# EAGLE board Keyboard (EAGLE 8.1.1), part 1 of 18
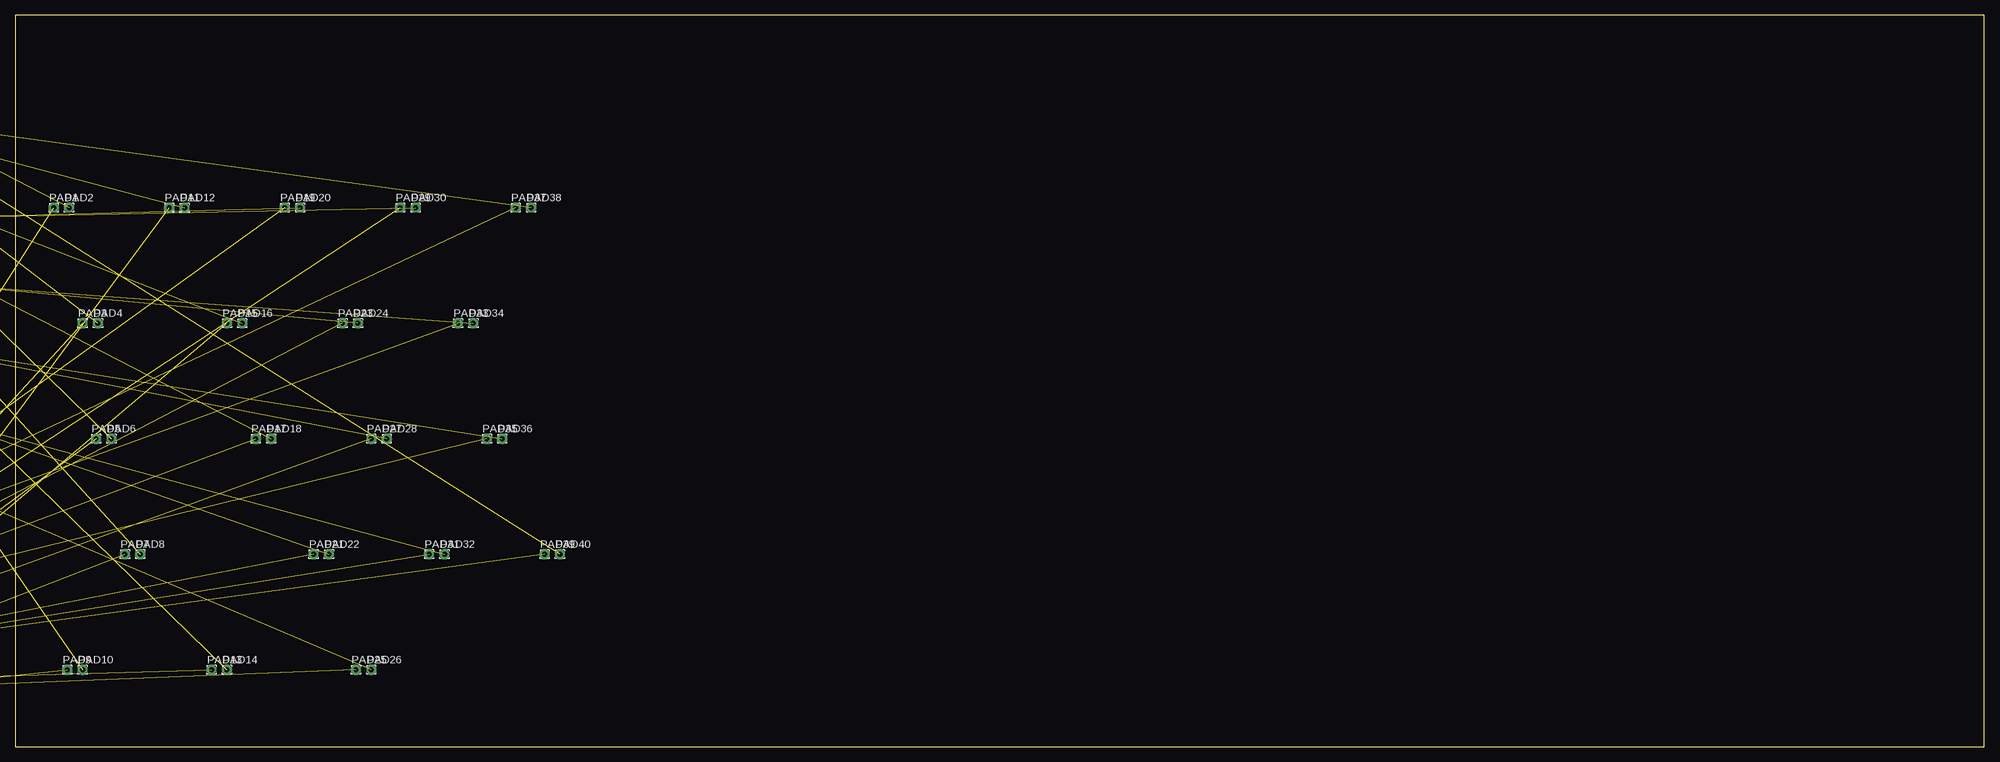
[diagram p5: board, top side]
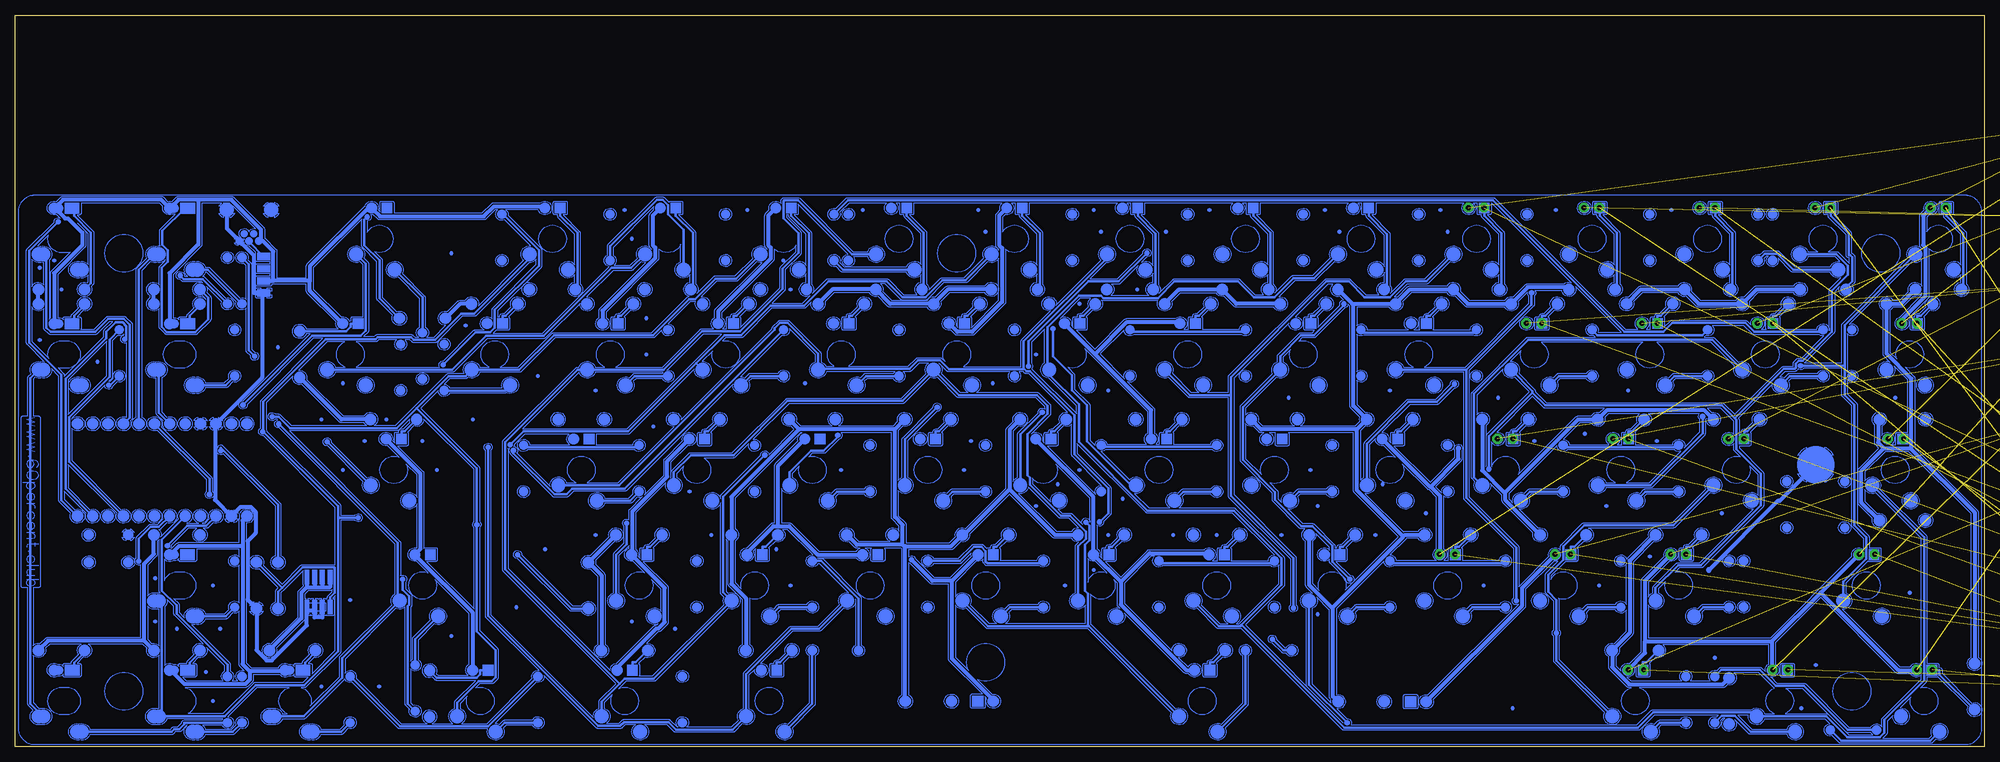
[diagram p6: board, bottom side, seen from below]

Size 324.79 x 120.64 mm. Coordinates in mm from the lower left corner, seen from the top.
Outline: 0,0 324.79,0 324.79,120.64 0,120.64 0,0
Copper layers (1*16): Top 0.035mm / dielectric 1.5mm / Bottom 0.035mm
Design rules "default": minimum track width 10mil, minimum drill 24mil, track to track 8mil, track to pad 8mil, pad to pad 8mil, via to via 8mil, smd to smd 8mil, copper to edge 40mil, drill to drill 8mil, minimum pad ring 10mil, minimum via ring 8mil, stop-mask expansion 4mil, vias tented up to drill 0mil, thermal gap 10mil

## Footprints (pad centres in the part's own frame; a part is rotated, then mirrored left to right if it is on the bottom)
2X5-SHROUDED = drill 1.016 pad 1.88: 1 -1.27,5.08; 2 1.27,5.08; 3 -1.27,2.54; 4 1.27,2.54; 5 -1.27,0; 6 1.27,0; 7 -1.27,-2.54; 8 1.27,-2.54; 9 -1.27,-5.08; 10 1.27,-5.08
1,6/0,8 = drill 0.813 pad 1.6 octagon: 1 0,0
R0805 = smd 1.3 x 1.5: 1 -0.95,0; 2 0.95,0
SOIC127P1030X265-20N = smd 1.981 x 0.559: 1 -4.674,5.715; 2 -4.674,4.445; 3 -4.674,3.175; 4 -4.674,1.905; 5 -4.674,0.635; 6 -4.674,-0.635; 7 -4.674,-1.905; 8 -4.674,-3.175; 9 -4.674,-4.445; 10 -4.674,-5.715; 11 4.674,-5.715; 12 4.674,-4.445; 13 4.674,-3.175; 14 4.674,-1.905; 15 4.674,-0.635; 16 4.674,0.635; 17 4.674,1.905; 18 4.674,3.175; 19 4.674,4.445; 20 4.674,5.715
SO14 = smd 0.6 x 1.2: 1 -3.81,-2.8; 2 -2.54,-2.8; 3 -1.27,-2.8; 4 0,-2.8; 5 1.27,-2.8; 6 2.54,-2.8; 7 3.81,-2.8; 8 3.81,2.8; 9 2.54,2.8; 10 1.27,2.8; 11 0,2.8; 12 -1.27,2.8; 13 -2.54,2.8; 14 -3.81,2.8
TEENSY_3.5/3.6 = drill 0.965: 0/RX -25.4,-7.62; 1/TX -22.86,-7.62; 2 -20.32,-7.62; 3/CANTX -17.78,-7.62; 3V3 7.62,-7.62; 3V3_2 17.78,-2.54; 3V3_LO -22.86,7.62; 4/CANRX -15.24,-7.62; 5 -12.7,-7.62; 6 -10.16,-7.62; 7 -7.62,-7.62; 8 -5.08,-7.62; 9/CS -2.54,-7.62; 10/CS 0,-7.62; 11/MOSI 2.54,-7.62; 12/MISO 5.08,-7.62; 13/SCK 5.08,7.62; 14/A0 2.54,7.62; 15/A1 0,7.62; 16/A2 -2.54,7.62; 17/A3 -5.08,7.62; 18/A4/SDA -7.62,7.62; 19/A5/SCL -10.16,7.62; 20/A6 -12.7,7.62; 21/A7 -15.24,7.62; 21/DAC0 12.7,7.62; 22/A8 -17.78,7.62; 23/A9 -20.32,7.62; 24 10.16,-7.62; 25 12.7,-7.62; 26 15.24,-7.62; 27 17.78,-7.62; 28 20.32,-7.62; 29 22.86,-7.62; 30 25.4,-7.62; 31/A12 27.94,-7.62; 32/A13 30.48,-7.62; 33/A14 30.48,7.62; 34/A15 27.94,7.62; 35/A16 25.4,7.62; 36/A17 22.86,7.62; 37/A18 20.32,7.62; 38/A19 17.78,7.62; 39/A20 15.24,7.62; A10 -17.78,5.08; A11 -15.24,5.08; A22/DAC1 10.16,7.62; AGND -25.4,7.62; AREF -20.32,5.08; GND -27.94,-7.62; GND2 7.62,7.62; GND3 17.78,0; PROG 17.78,2.54; RESET 17.78,5.08; U5V -21.59,-4.445; UD+ -16.51,-4.445; UD- -19.05,-4.445; UGND1 -13.97,-4.445; UGND2 -11.43,-4.445; VBAT 17.78,-5.08; VIN -27.94,7.62; VUSB -25.4,5.08

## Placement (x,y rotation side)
J1  [2X5-SHROUDED]  not placed on the board
PAD1  [1,6/0,8]  6.35,88.9 0 top
PAD2  [1,6/0,8]  8.89,88.9 0 top
PAD3  [1,6/0,8]  11.11,69.85 0 top
PAD4  [1,6/0,8]  13.65,69.85 0 top
PAD5  [1,6/0,8]  13.34,50.8 0 top
PAD6  [1,6/0,8]  15.88,50.8 0 top
PAD7  [1,6/0,8]  18.1,31.75 0 top
PAD8  [1,6/0,8]  20.64,31.75 0 top
PAD9  [1,6/0,8]  8.57,12.7 0 top
PAD10  [1,6/0,8]  11.11,12.7 0 top
PAD11  [1,6/0,8]  25.4,88.9 0 top
PAD12  [1,6/0,8]  27.94,88.9 0 top
PAD13  [1,6/0,8]  32.38,12.7 0 top
PAD14  [1,6/0,8]  34.92,12.7 0 top
PAD15  [1,6/0,8]  34.92,69.85 0 top
PAD16  [1,6/0,8]  37.47,69.85 0 top
PAD17  [1,6/0,8]  39.69,50.8 0 top
PAD18  [1,6/0,8]  42.23,50.8 0 top
PAD19  [1,6/0,8]  44.45,88.9 0 top
PAD20  [1,6/0,8]  46.99,88.9 0 top
PAD21  [1,6/0,8]  49.21,31.75 0 top
PAD22  [1,6/0,8]  51.75,31.75 0 top
PAD23  [1,6/0,8]  53.98,69.85 0 top
PAD24  [1,6/0,8]  56.52,69.85 0 top
PAD25  [1,6/0,8]  56.2,12.7 0 top
PAD26  [1,6/0,8]  58.74,12.7 0 top
PAD27  [1,6/0,8]  58.74,50.8 0 top
PAD28  [1,6/0,8]  61.28,50.8 0 top
PAD29  [1,6/0,8]  63.5,88.9 0 top
PAD30  [1,6/0,8]  66.04,88.9 0 top
PAD31  [1,6/0,8]  68.26,31.75 0 top
PAD32  [1,6/0,8]  70.8,31.75 0 top
PAD33  [1,6/0,8]  73.03,69.85 0 top
PAD34  [1,6/0,8]  75.56,69.85 0 top
PAD35  [1,6/0,8]  77.79,50.8 0 top
PAD36  [1,6/0,8]  80.33,50.8 0 top
PAD37  [1,6/0,8]  82.55,88.9 0 top
PAD38  [1,6/0,8]  85.09,88.9 0 top
PAD39  [1,6/0,8]  87.31,31.75 0 top
PAD40  [1,6/0,8]  89.85,31.75 0 top
PAD41  [1,6/0,8]  not placed on the board
PAD42  [1,6/0,8]  not placed on the board
PAD43  [1,6/0,8]  not placed on the board
PAD44  [1,6/0,8]  not placed on the board
PAD45  [1,6/0,8]  not placed on the board
PAD46  [1,6/0,8]  not placed on the board
PAD47  [1,6/0,8]  not placed on the board
PAD48  [1,6/0,8]  not placed on the board
PAD49  [1,6/0,8]  not placed on the board
PAD50  [1,6/0,8]  not placed on the board
PAD51  [1,6/0,8]  not placed on the board
PAD52  [1,6/0,8]  not placed on the board
PAD53  [1,6/0,8]  not placed on the board
PAD54  [1,6/0,8]  not placed on the board
PAD55  [1,6/0,8]  not placed on the board
PAD56  [1,6/0,8]  not placed on the board
PAD57  [1,6/0,8]  not placed on the board
PAD58  [1,6/0,8]  not placed on the board
PAD59  [1,6/0,8]  not placed on the board
PAD60  [1,6/0,8]  not placed on the board
PAD61  [1,6/0,8]  not placed on the board
PAD62  [1,6/0,8]  not placed on the board
PAD63  [1,6/0,8]  not placed on the board
PAD64  [1,6/0,8]  not placed on the board
PAD65  [1,6/0,8]  not placed on the board
PAD66  [1,6/0,8]  not placed on the board
PAD67  [1,6/0,8]  not placed on the board
PAD68  [1,6/0,8]  not placed on the board
PAD69  [1,6/0,8]  not placed on the board
PAD70  [1,6/0,8]  not placed on the board
PAD71  [1,6/0,8]  not placed on the board
PAD72  [1,6/0,8]  not placed on the board
PAD73  [1,6/0,8]  not placed on the board
PAD74  [1,6/0,8]  not placed on the board
PAD75  [1,6/0,8]  not placed on the board
PAD76  [1,6/0,8]  not placed on the board
PAD77  [1,6/0,8]  not placed on the board
PAD78  [1,6/0,8]  not placed on the board
PAD79  [1,6/0,8]  not placed on the board
PAD80  [1,6/0,8]  not placed on the board
PAD81  [1,6/0,8]  not placed on the board
PAD82  [1,6/0,8]  not placed on the board
PAD83  [1,6/0,8]  not placed on the board
PAD84  [1,6/0,8]  not placed on the board
PAD85  [1,6/0,8]  not placed on the board
PAD86  [1,6/0,8]  not placed on the board
PAD87  [1,6/0,8]  not placed on the board
PAD88  [1,6/0,8]  not placed on the board
PAD89  [1,6/0,8]  not placed on the board
PAD90  [1,6/0,8]  not placed on the board
PAD91  [1,6/0,8]  not placed on the board
PAD92  [1,6/0,8]  not placed on the board
PAD93  [1,6/0,8]  not placed on the board
PAD94  [1,6/0,8]  not placed on the board
PAD95  [1,6/0,8]  not placed on the board
PAD96  [1,6/0,8]  not placed on the board
PAD97  [1,6/0,8]  not placed on the board
PAD98  [1,6/0,8]  not placed on the board
PAD99  [1,6/0,8]  not placed on the board
PAD100  [1,6/0,8]  not placed on the board
PAD101  [1,6/0,8]  not placed on the board
PAD102  [1,6/0,8]  not placed on the board
PAD103  [1,6/0,8]  not placed on the board
PAD104  [1,6/0,8]  not placed on the board
PAD105  [1,6/0,8]  not placed on the board
PAD106  [1,6/0,8]  not placed on the board
PAD107  [1,6/0,8]  not placed on the board
PAD108  [1,6/0,8]  not placed on the board
PAD109  [1,6/0,8]  not placed on the board
PAD110  [1,6/0,8]  not placed on the board
PAD111  [1,6/0,8]  not placed on the board
PAD112  [1,6/0,8]  not placed on the board
PAD113  [1,6/0,8]  not placed on the board
PAD114  [1,6/0,8]  not placed on the board
PAD115  [1,6/0,8]  not placed on the board
PAD116  [1,6/0,8]  not placed on the board
PAD117  [1,6/0,8]  not placed on the board
PAD118  [1,6/0,8]  not placed on the board
PAD119  [1,6/0,8]  not placed on the board
PAD120  [1,6/0,8]  not placed on the board
PAD121  [1,6/0,8]  not placed on the board
PAD122  [1,6/0,8]  not placed on the board
PAD123  [1,6/0,8]  not placed on the board
PAD124  [1,6/0,8]  not placed on the board
PAD125  [1,6/0,8]  not placed on the board
PAD126  [1,6/0,8]  not placed on the board
PAD127  [1,6/0,8]  not placed on the board
PAD128  [1,6/0,8]  not placed on the board
PAD129  [1,6/0,8]  not placed on the board
PAD130  [1,6/0,8]  not placed on the board
PAD131  [1,6/0,8]  not placed on the board
PAD132  [1,6/0,8]  not placed on the board
PAD133  [1,6/0,8]  not placed on the board
PAD134  [1,6/0,8]  not placed on the board
PAD135  [1,6/0,8]  not placed on the board
PAD136  [1,6/0,8]  not placed on the board
PAD137  [1,6/0,8]  not placed on the board
PAD138  [1,6/0,8]  not placed on the board
R1  [R0805]  not placed on the board
R2  [R0805]  not placed on the board
R3  [R0805]  not placed on the board
R4  [R0805]  not placed on the board
R5  [R0805]  not placed on the board
R5V  [R0805]  not placed on the board
R6  [R0805]  not placed on the board
R7  [R0805]  not placed on the board
R8  [R0805]  not placed on the board
R9  [R0805]  not placed on the board
R10  [R0805]  not placed on the board
R11  [R0805]  not placed on the board
R12  [R0805]  not placed on the board
R13  [R0805]  not placed on the board
R14  [R0805]  not placed on the board
R15  [R0805]  not placed on the board
R16  [R0805]  not placed on the board
R17  [R0805]  not placed on the board
R18  [R0805]  not placed on the board
R19  [R0805]  not placed on the board
R20  [R0805]  not placed on the board
R21  [R0805]  not placed on the board
R22  [R0805]  not placed on the board
R23  [R0805]  not placed on the board
R24  [R0805]  not placed on the board
R25  [R0805]  not placed on the board
R26  [R0805]  not placed on the board
R27  [R0805]  not placed on the board
R28  [R0805]  not placed on the board
R29  [R0805]  not placed on the board
R30  [R0805]  not placed on the board
R31  [R0805]  not placed on the board
R32  [R0805]  not placed on the board
R33  [R0805]  not placed on the board
R34  [R0805]  not placed on the board
R35  [R0805]  not placed on the board
R36  [R0805]  not placed on the board
R37  [R0805]  not placed on the board
R38  [R0805]  not placed on the board
R39  [R0805]  not placed on the board
R40  [R0805]  not placed on the board
R41  [R0805]  not placed on the board
R42  [R0805]  not placed on the board
R43  [R0805]  not placed on the board
R44  [R0805]  not placed on the board
R45  [R0805]  not placed on the board
R46  [R0805]  not placed on the board
R47  [R0805]  not placed on the board
R48  [R0805]  not placed on the board
R49  [R0805]  not placed on the board
R50  [R0805]  not placed on the board
R51  [R0805]  not placed on the board
R52  [R0805]  not placed on the board
R53  [R0805]  not placed on the board
R54  [R0805]  not placed on the board
R55  [R0805]  not placed on the board
R56  [R0805]  not placed on the board
R57  [R0805]  not placed on the board
R58  [R0805]  not placed on the board
R59  [R0805]  not placed on the board
R60  [R0805]  not placed on the board
R61  [R0805]  not placed on the board
R62  [R0805]  not placed on the board
R63  [R0805]  not placed on the board
R64  [R0805]  not placed on the board
R65  [R0805]  not placed on the board
R66  [R0805]  not placed on the board
R67  [R0805]  not placed on the board
R68  [R0805]  not placed on the board
R69  [R0805]  not placed on the board
RG  [R0805]  not placed on the board
U1  TPIC6B595DW  [SOIC127P1030X265-20N]  not placed on the board
U2  TPIC6B595DW  [SOIC127P1030X265-20N]  not placed on the board
U3  TPIC6B595DW  [SOIC127P1030X265-20N]  not placed on the board
U4  TPIC6B595DW  [SOIC127P1030X265-20N]  not placed on the board
U5  TPIC6B595DW  [SOIC127P1030X265-20N]  not placed on the board
U6  TPIC6B595DW  [SOIC127P1030X265-20N]  not placed on the board
U7  TPIC6B595DW  [SOIC127P1030X265-20N]  not placed on the board
U8  TPIC6B595DW  [SOIC127P1030X265-20N]  not placed on the board
U9  TPIC6B595DW  [SOIC127P1030X265-20N]  not placed on the board
U10  TPIC6B595DW  [SOIC127P1030X265-20N]  not placed on the board
U11  TPIC6B595DW  [SOIC127P1030X265-20N]  not placed on the board
U12  TPIC6B595DW  [SOIC127P1030X265-20N]  not placed on the board
U13  TPIC6B595DW  [SOIC127P1030X265-20N]  not placed on the board
U14  TPIC6B595DW  [SOIC127P1030X265-20N]  not placed on the board
U15  TPIC6B595DW  [SOIC127P1030X265-20N]  not placed on the board
U16  TPIC6B595DW  [SOIC127P1030X265-20N]  not placed on the board
U17  TPIC6B595DW  [SOIC127P1030X265-20N]  not placed on the board
U18  TPIC6B595DW  [SOIC127P1030X265-20N]  not placed on the board
U19  [SO14]  not placed on the board
U$59  TEENSY_3.5/3.6  [TEENSY_3.5/3.6]  not placed on the board

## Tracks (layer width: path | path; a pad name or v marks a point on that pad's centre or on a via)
N$1  (1 unrouted)
N$2  (1 unrouted)
N$3  (36 unrouted)
N$4  (1 unrouted)
N$5  (1 unrouted)
N$6  (1 unrouted)
N$7  (1 unrouted)
N$8  (1 unrouted)
N$9  (1 unrouted)
N$10  (1 unrouted)
N$11  (1 unrouted)
N$12  (18 unrouted)
N$13  (1 unrouted)
N$14  (1 unrouted)
N$15  (1 unrouted)
N$16  (1 unrouted)
N$17  (1 unrouted)
N$18  (1 unrouted)
N$19  (1 unrouted)
N$20  (1 unrouted)
N$21  (1 unrouted)
N$22  (1 unrouted)
N$23  (1 unrouted)
N$24  (1 unrouted)
N$25  (1 unrouted)
N$26  (1 unrouted)
N$27  (1 unrouted)
N$28  (1 unrouted)
N$29  (1 unrouted)
N$30  (1 unrouted)
N$31  (1 unrouted)
N$32  (1 unrouted)
N$33  (1 unrouted)
N$34  (1 unrouted)
N$35  (1 unrouted)
N$36  (1 unrouted)
N$37  (1 unrouted)
N$38  (1 unrouted)
N$39  (1 unrouted)
N$40  (1 unrouted)
N$41  (1 unrouted)
N$42  (1 unrouted)
N$43  (1 unrouted)
N$44  (1 unrouted)
N$45  (1 unrouted)
N$46  (1 unrouted)
N$47  (1 unrouted)
N$48  (1 unrouted)
N$49  (1 unrouted)
N$50  (1 unrouted)
N$51  (1 unrouted)
N$52  (1 unrouted)
N$53  (1 unrouted)
N$54  (1 unrouted)
N$55  (1 unrouted)
N$56  (1 unrouted)
N$57  (1 unrouted)
N$58  (1 unrouted)
N$59  (1 unrouted)
N$60  (1 unrouted)
N$61  (20 unrouted)
N$62  (1 unrouted)
N$63  (19 unrouted)
N$64  (1 unrouted)
N$65  (1 unrouted)
N$66  (1 unrouted)
N$67  (1 unrouted)
N$68  (1 unrouted)
N$69  (1 unrouted)
N$70  (1 unrouted)
N$71  (1 unrouted)
N$72  (1 unrouted)
N$73  (1 unrouted)
N$74  (1 unrouted)
N$75  (1 unrouted)
N$76  (1 unrouted)
N$77  (1 unrouted)
N$78  (1 unrouted)
N$79  (1 unrouted)
N$80  (1 unrouted)
N$81  (1 unrouted)
N$82  (1 unrouted)
N$83  (1 unrouted)
N$84  (1 unrouted)
N$85  (1 unrouted)
N$86  (1 unrouted)
N$87  (1 unrouted)
N$88  (1 unrouted)
N$89  (1 unrouted)
N$90  (1 unrouted)
N$91  (1 unrouted)
N$92  (1 unrouted)
N$93  (1 unrouted)
N$94  (1 unrouted)
N$95  (56 unrouted)
N$96  (1 unrouted)
N$97  (1 unrouted)
N$98  (1 unrouted)
N$99  (1 unrouted)
N$100  (1 unrouted)
N$101  (1 unrouted)
N$102  (1 unrouted)
N$103  (1 unrouted)
N$104  (1 unrouted)
N$105  (1 unrouted)
N$106  (1 unrouted)
N$107  (1 unrouted)
N$108  (1 unrouted)
N$109  (1 unrouted)
N$110  (1 unrouted)
N$111  (1 unrouted)
N$112  (1 unrouted)
N$113  (1 unrouted)
N$114  (1 unrouted)
N$115  (1 unrouted)
N$116  (1 unrouted)
N$117  (1 unrouted)
N$118  (1 unrouted)
N$119  (1 unrouted)
N$120  (1 unrouted)
N$121  (1 unrouted)
N$122  (1 unrouted)
N$123  (1 unrouted)
N$124  (1 unrouted)
N$125  (1 unrouted)
N$126  (1 unrouted)
N$127  (1 unrouted)
N$128  (1 unrouted)
N$129  (1 unrouted)
N$130  (1 unrouted)
N$131  (1 unrouted)
N$132  (1 unrouted)
N$133  (1 unrouted)
N$134  (1 unrouted)
N$135  (1 unrouted)
N$136  (1 unrouted)
N$137  (1 unrouted)
N$138  (1 unrouted)
N$139  (1 unrouted)
N$140  (1 unrouted)
N$141  (1 unrouted)
N$142  (1 unrouted)
N$143  (1 unrouted)
N$144  (1 unrouted)
N$145  (1 unrouted)
N$146  (1 unrouted)
N$147  (1 unrouted)
N$148  (1 unrouted)
N$149  (1 unrouted)
N$150  (1 unrouted)
N$151  (1 unrouted)
N$152  (1 unrouted)
N$153  (1 unrouted)
N$154  (1 unrouted)
N$155  (1 unrouted)
N$156  (1 unrouted)
N$157  (1 unrouted)
N$158  (1 unrouted)
N$159  (1 unrouted)
N$160  (1 unrouted)
N$161  (1 unrouted)
N$162  (1 unrouted)
N$163  (1 unrouted)
N$164  (1 unrouted)
N$165  (1 unrouted)
N$166  (1 unrouted)
N$167  (1 unrouted)
N$168  (1 unrouted)
N$169  (1 unrouted)
N$170  (1 unrouted)
N$171  (1 unrouted)
N$172  (1 unrouted)
N$173  (1 unrouted)
N$174  (1 unrouted)
N$175  (1 unrouted)
N$176  (1 unrouted)
N$177  (1 unrouted)
N$178  (1 unrouted)
N$179  (1 unrouted)
N$180  (1 unrouted)
N$181  (1 unrouted)
N$182  (1 unrouted)
N$183  (1 unrouted)
N$184  (1 unrouted)
N$185  (1 unrouted)
N$186  (1 unrouted)
N$187  (1 unrouted)
N$188  (1 unrouted)
N$189  (1 unrouted)
N$190  (1 unrouted)
N$191  (1 unrouted)
N$192  (1 unrouted)
N$193  (1 unrouted)
N$194  (1 unrouted)
N$195  (1 unrouted)
N$196  (1 unrouted)
N$197  (1 unrouted)
N$198  (1 unrouted)
N$199  (1 unrouted)
N$200  (1 unrouted)
N$201  (1 unrouted)
N$202  (1 unrouted)
N$203  (1 unrouted)
N$204  (1 unrouted)
N$205  (1 unrouted)
N$206  (1 unrouted)
N$207  (1 unrouted)
N$208  (1 unrouted)
N$209  (1 unrouted)
N$210  (1 unrouted)
N$211  (1 unrouted)
N$212  (1 unrouted)
N$213  (1 unrouted)
N$214  (1 unrouted)
N$215  (1 unrouted)
N$216  (1 unrouted)
N$217  (1 unrouted)
N$218  (1 unrouted)
N$219  (1 unrouted)
N$220  (1 unrouted)
N$221  (1 unrouted)
N$222  (1 unrouted)
N$223  (1 unrouted)
N$224  (1 unrouted)
N$225  (1 unrouted)
N$226  (1 unrouted)
N$227  (1 unrouted)
N$228  (1 unrouted)
N$229  (1 unrouted)
N$230  (1 unrouted)
N$231  (1 unrouted)
N$232  (1 unrouted)
N$233  (1 unrouted)
N$234  (1 unrouted)
N$235  (1 unrouted)
N$236  (1 unrouted)
N$237  (1 unrouted)
N$238  (1 unrouted)
N$239  (1 unrouted)
N$240  (1 unrouted)
N$241  (1 unrouted)
N$242  (1 unrouted)
N$243  (1 unrouted)
N$244  (1 unrouted)
S$1
  Bottom 0: 2.79,0.4 2.62,0.44
S$2
  Bottom 0: 2.62,0.44 2.44,0.48
S$3
  Bottom 0: 2.44,0.48 2.27,0.54
S$4
  Bottom 0: 2.27,0.54 2.11,0.6
S$5
  Bottom 0: 2.11,0.6 1.94,0.68
S$6
  Bottom 0: 1.94,0.68 1.78,0.77
S$7
  Bottom 0: 1.78,0.77 1.63,0.86
S$8
  Bottom 0: 1.63,0.86 1.49,0.97
S$9
  Bottom 0: 1.49,0.97 1.35,1.08
S$10
  Bottom 0: 1.35,1.08 1.22,1.2
S$11
  Bottom 0: 1.22,1.2 1.09,1.33
S$12
  Bottom 0: 1.09,1.33 0.98,1.47
S$13
  Bottom 0: 0.98,1.47 0.87,1.62
S$14
  Bottom 0: 0.87,1.62 0.78,1.76
S$15
  Bottom 0: 0.78,1.76 0.69,1.92
S$16
  Bottom 0: 0.69,1.92 0.62,2.08
S$17
  Bottom 0: 0.62,2.08 0.55,2.25
S$18
  Bottom 0: 0.55,2.25 0.49,2.43
S$19
  Bottom 0: 0.49,2.43 0.45,2.6
S$20
  Bottom 0: 0.45,2.6 0.41,2.77
S$21
  Bottom 0: 0.41,2.77 0.41,2.8
S$22
  Bottom 0: 0.41,2.8 0.41,87.33
S$23
  Bottom 0: 0.41,87.33 0.41,88.52
S$24
  Bottom 0: 0.41,88.52 0.45,88.69
S$25
  Bottom 0: 0.45,88.69 0.49,88.87
S$26
  Bottom 0: 0.49,88.87 0.54,89.04
S$27
  Bottom 0: 0.54,89.04 0.61,89.21
S$28
  Bottom 0: 0.61,89.21 0.69,89.37
S$29
  Bottom 0: 0.69,89.37 0.77,89.53
S$30
  Bottom 0: 0.77,89.53 0.87,89.68
S$31
  Bottom 0: 0.87,89.68 0.97,89.82
S$32
  Bottom 0: 0.97,89.82 1.08,89.96
S$33
  Bottom 0: 1.08,89.96 1.21,90.09
S$34
  Bottom 0: 1.21,90.09 1.34,90.21
S$35
  Bottom 0: 1.34,90.21 1.48,90.33
S$36
  Bottom 0: 1.48,90.33 1.62,90.44
S$37
  Bottom 0: 1.62,90.44 1.77,90.53
S$38
  Bottom 0: 1.77,90.53 1.93,90.62
S$39
  Bottom 0: 1.93,90.62 2.09,90.7
S$40
  Bottom 0: 2.09,90.7 2.26,90.76
S$41
  Bottom 0: 2.26,90.76 2.43,90.82
S$42
  Bottom 0: 2.43,90.82 2.6,90.86
S$43
  Bottom 0: 2.6,90.86 2.78,90.9
S$44
  Bottom 0: 2.78,90.9 2.79,90.9
S$45
  Bottom 0: 2.79,90.9
S$46
  Bottom 0: 2.79,90.9 321.91,90.9
S$47
  Bottom 0: 321.91,90.9
S$48
  Bottom 0: 321.91,90.9 322.09,90.87
S$49
  Bottom 0: 322.09,90.87 322.26,90.82
S$50
  Bottom 0: 322.26,90.82 322.44,90.77
S$51
  Bottom 0: 322.44,90.77 322.6,90.7
S$52
  Bottom 0: 322.6,90.7 322.76,90.62
S$53
  Bottom 0: 322.76,90.62 322.92,90.54
S$54
  Bottom 0: 322.92,90.54 323.07,90.45
S$55
  Bottom 0: 323.07,90.45 323.22,90.34
S$56
  Bottom 0: 323.22,90.34 323.36,90.23
S$57
  Bottom 0: 323.36,90.23 323.49,90.1
S$58
  Bottom 0: 323.49,90.1 323.61,89.97
S$59
  Bottom 0: 323.61,89.97 323.73,89.84
S$60
  Bottom 0: 323.73,89.84 323.83,89.69
S$61
  Bottom 0: 323.83,89.69 323.93,89.54
S$62
  Bottom 0: 323.93,89.54 324.01,89.38
S$63
  Bottom 0: 324.01,89.38 324.09,89.22
S$64
  Bottom 0: 324.09,89.22 324.16,89.06
S$65
  Bottom 0: 324.16,89.06 324.21,88.88
S$66
  Bottom 0: 324.21,88.88 324.26,88.71
S$67
  Bottom 0: 324.26,88.71 324.3,88.54
S$68
  Bottom 0: 324.3,88.54 324.3,2.79
S$69
  Bottom 0: 324.3,2.79 324.26,2.61
S$70
  Bottom 0: 324.26,2.61 324.22,2.44
S$71
  Bottom 0: 324.22,2.44 324.16,2.27
S$72
  Bottom 0: 324.16,2.27 324.1,2.1
S$73
  Bottom 0: 324.1,2.1 324.02,1.94
S$74
  Bottom 0: 324.02,1.94 323.94,1.78
S$75
  Bottom 0: 323.94,1.78 323.84,1.63
S$76
  Bottom 0: 323.84,1.63 323.74,1.48
S$77
  Bottom 0: 323.74,1.48 323.62,1.34
S$78
  Bottom 0: 323.62,1.34 323.49,1.21
S$79
  Bottom 0: 323.49,1.21 323.37,1.09
S$80
  Bottom 0: 323.37,1.09 323.23,0.98
S$81
  Bottom 0: 323.23,0.98 323.08,0.87
S$82
  Bottom 0: 323.08,0.87 322.93,0.78
S$83
  Bottom 0: 322.93,0.78 322.78,0.69
S$84
  Bottom 0: 322.78,0.69 322.62,0.61
S$85
  Bottom 0: 322.62,0.61 322.45,0.54
S$86
  Bottom 0: 322.45,0.54 322.28,0.48
S$87
  Bottom 0: 322.28,0.48 322.11,0.44
S$88
  Bottom 0: 322.11,0.44 321.93,0.41
S$89
  Bottom 0: 321.93,0.41 321.91,0.4
S$90
  Bottom 0: 321.91,0.4 2.79,0.4
S$91
  Bottom 0: 8.88,0.55 23.62,0.55
S$92
  Bottom 0: 23.62,0.55 23.69,0.55
S$93
  Bottom 0: 23.69,0.55 23.75,0.57
S$94
  Bottom 0: 23.75,0.57 23.82,0.59
S$95
  Bottom 0: 23.82,0.59 23.88,0.63
S$96
  Bottom 0: 23.88,0.63 23.93,0.67
S$97
  Bottom 0: 23.93,0.67 25.09,1.83
S$98
  Bottom 0: 25.09,1.83 25.19,1.8
S$99
  Bottom 0: 25.19,1.8 25.49,1.77
S$100
  Bottom 0: 25.49,1.77 25.79,1.84
S$101
  Bottom 0: 25.79,1.84 26.05,1.99
S$102
  Bottom 0: 26.05,1.99 26.26,2.21
S$103
  Bottom 0: 26.26,2.21 26.39,2.49
S$104
  Bottom 0: 26.39,2.49 26.43,2.79
S$105
  Bottom 0: 26.43,2.79 26.39,3.09
S$106
  Bottom 0: 26.39,3.09 26.26,3.36
S$107
  Bottom 0: 26.26,3.36 26.05,3.58
S$108
  Bottom 0: 26.05,3.58 25.79,3.73
S$109
  Bottom 0: 25.79,3.73 25.49,3.8
S$110
  Bottom 0: 25.49,3.8 25.46,3.79
S$111
  Bottom 0: 25.46,3.79 26.24,4.58
S$112
  Bottom 0: 26.24,4.58 36.24,4.58
S$113
  Bottom 0: 36.24,4.58 36.26,4.5
S$114
  Bottom 0: 36.26,4.5 36.43,4.19
S$115
  Bottom 0: 36.43,4.19 36.67,3.94
S$116
  Bottom 0: 36.67,3.94 36.96,3.75
S$117
  Bottom 0: 36.96,3.75 37.3,3.65
S$118
  Bottom 0: 37.3,3.65 37.65,3.62
S$119
  Bottom 0: 37.65,3.62 37.99,3.69
S$120
  Bottom 0: 37.99,3.69 38.3,3.84
S$121
  Bottom 0: 38.3,3.84 38.58,4.06
S$122
  Bottom 0: 38.58,4.06 38.78,4.35
S$123
  Bottom 0: 38.78,4.35 38.91,4.67
S$124
  Bottom 0: 38.91,4.67 38.96,5.02
S$125
  Bottom 0: 38.96,5.02 38.92,5.23
S$126
  Bottom 0: 38.92,5.23 40.66,5.23
S$127
  Bottom 0: 40.66,5.23 38.35,2.92
S$128
  Bottom 0: 38.35,2.92 32.52,2.92
S$129
  Bottom 0: 32.52,2.92 32.43,3.15
S$130
  Bottom 0: 32.43,3.15 32.23,3.43
S$131
  Bottom 0: 32.23,3.43 31.96,3.65
S$132
  Bottom 0: 31.96,3.65 31.64,3.81
S$133
  Bottom 0: 31.64,3.81 31.29,3.87
S$134
  Bottom 0: 31.29,3.87 30.94,3.85
S$135
  Bottom 0: 30.94,3.85 30.61,3.74
S$136
  Bottom 0: 30.61,3.74 30.32,3.55
S$137
  Bottom 0: 30.32,3.55 30.08,3.3
S$138
  Bottom 0: 30.08,3.3 29.91,2.99
S$139
  Bottom 0: 29.91,2.99 29.82,2.65
S$140
  Bottom 0: 29.82,2.65 29.82,2.3
S$141
  Bottom 0: 29.82,2.3 29.91,1.96
S$142
  Bottom 0: 29.91,1.96 30.08,1.65
S$143
  Bottom 0: 30.08,1.65 30.32,1.4
S$144
  Bottom 0: 30.32,1.4 30.61,1.21
S$145
  Bottom 0: 30.61,1.21 30.94,1.1
S$146
  Bottom 0: 30.94,1.1 31.29,1.08
S$147
  Bottom 0: 31.29,1.08 31.64,1.15
S$148
  Bottom 0: 31.64,1.15 31.96,1.3
S$149
  Bottom 0: 31.96,1.3 32.23,1.52
S$150
  Bottom 0: 32.23,1.52 32.43,1.81
S$151
  Bottom 0: 32.43,1.81 32.52,2.04
S$152
  Bottom 0: 32.52,2.04 38.53,2.04
S$153
  Bottom 0: 38.53,2.04 38.6,2.04
S$154
  Bottom 0: 38.6,2.04 38.67,2.06
S$155
  Bottom 0: 38.67,2.06 38.73,2.08
S$156
  Bottom 0: 38.73,2.08 38.79,2.12
S$157
  Bottom 0: 38.79,2.12 38.85,2.16
S$158
  Bottom 0: 38.85,2.16 41.14,4.45
S$159
  Bottom 0: 41.14,4.45 40.99,4.22
S$160
  Bottom 0: 40.99,4.22 40.9,3.9
S$161
  Bottom 0: 40.9,3.9 40.9,3.58
S$162
  Bottom 0: 40.9,3.58 40.99,3.26
S$163
  Bottom 0: 40.99,3.26 41.17,2.99
S$164
  Bottom 0: 41.17,2.99 41.4,2.77
S$165
  Bottom 0: 41.4,2.77 41.69,2.62
S$166
  Bottom 0: 41.69,2.62 42.01,2.55
S$167
  Bottom 0: 42.01,2.55 42.33,2.57
S$168
  Bottom 0: 42.33,2.57 42.64,2.68
S$169
  Bottom 0: 42.64,2.68 42.9,2.87
S$170
  Bottom 0: 42.9,2.87 43.11,3.12
S$171
  Bottom 0: 43.11,3.12 43.24,3.42
S$172
  Bottom 0: 43.24,3.42 43.28,3.74
S$173
  Bottom 0: 43.28,3.74 43.24,4.06
S$174
  Bottom 0: 43.24,4.06 43.11,4.36
S$175
  Bottom 0: 43.11,4.36 42.9,4.62
S$176
  Bottom 0: 42.9,4.62 42.83,4.67
S$177
  Bottom 0: 42.83,4.67 43.15,4.67
S$178
  Bottom 0: 43.15,4.67 43.52,4.3
S$179
  Bottom 0: 43.52,4.3 43.46,4.13
S$180
  Bottom 0: 43.46,4.13 43.46,3.82
S$181
  Bottom 0: 43.46,3.82 43.55,3.53
S$182
  Bottom 0: 43.55,3.53 43.72,3.28
S$183
  Bottom 0: 43.72,3.28 43.96,3.1
S$184
  Bottom 0: 43.96,3.1 44.24,2.98
S$185
  Bottom 0: 44.24,2.98 44.54,2.96
S$186
  Bottom 0: 44.54,2.96 44.84,3.03
S$187
  Bottom 0: 44.84,3.03 45.1,3.18
S$188
  Bottom 0: 45.1,3.18 45.31,3.4
S$189
  Bottom 0: 45.31,3.4 45.44,3.67
S$190
  Bottom 0: 45.44,3.67 45.48,3.98
S$191
  Bottom 0: 45.48,3.98 45.44,4.28
S$192
  Bottom 0: 45.44,4.28 45.31,4.55
S$193
  Bottom 0: 45.31,4.55 45.1,4.77
S$194
  Bottom 0: 45.1,4.77 44.84,4.92
S$195
  Bottom 0: 44.84,4.92 44.54,4.99
S$196
  Bottom 0: 44.54,4.99 44.24,4.97
S$197
  Bottom 0: 44.24,4.97 44.14,4.92
S$198
  Bottom 0: 44.14,4.92 43.84,5.23
S$199
  Bottom 0: 43.84,5.23 54.41,5.23
S$200
  Bottom 0: 54.41,5.23 56.8,2.84
S$201
  Bottom 0: 56.8,2.84 56.85,2.8
S$202
  Bottom 0: 56.85,2.8 56.91,2.76
S$203
  Bottom 0: 56.91,2.76 56.97,2.74
S$204
  Bottom 0: 56.97,2.74 57.04,2.72
S$205
  Bottom 0: 57.04,2.72 57.11,2.71
S$206
  Bottom 0: 57.11,2.71 105.56,2.71
S$207
  Bottom 0: 105.56,2.71 105.64,2.72
S$208
  Bottom 0: 105.64,2.72 105.7,2.74
S$209
  Bottom 0: 105.7,2.74 105.76,2.76
S$210
  Bottom 0: 105.76,2.76 105.82,2.8
S$211
  Bottom 0: 105.82,2.8 105.88,2.84
S$212
  Bottom 0: 105.88,2.84 122.52,19.48
S$213
  Bottom 0: 122.52,19.48 122.58,19.46
S$214
  Bottom 0: 122.58,19.46 122.64,19.44
S$215
  Bottom 0: 122.64,19.44 122.72,19.44
S$216
  Bottom 0: 122.72,19.44 126.24,19.44
S$217
  Bottom 0: 126.24,19.44 126.31,19.44
S$218
  Bottom 0: 126.31,19.44 126.38,19.46
S$219
  Bottom 0: 126.38,19.46 126.44,19.48
S$220
  Bottom 0: 126.44,19.48 126.5,19.52
S$221
  Bottom 0: 126.5,19.52 126.56,19.57
S$222
  Bottom 0: 126.56,19.57 129.8,22.82
S$223
  Bottom 0: 129.8,22.82 129.83,22.8
S$224
  Bottom 0: 129.83,22.8 130.16,22.7
S$225
  Bottom 0: 130.16,22.7 130.51,22.68
S$226
  Bottom 0: 130.51,22.68 130.86,22.74
S$227
  Bottom 0: 130.86,22.74 131.17,22.89
S$228
  Bottom 0: 131.17,22.89 131.44,23.11
S$229
  Bottom 0: 131.44,23.11 131.65,23.4
S$230
  Bottom 0: 131.65,23.4 131.78,23.72
S$231
  Bottom 0: 131.78,23.72 131.82,24.07
S$232
  Bottom 0: 131.82,24.07 131.78,24.41
S$233
  Bottom 0: 131.78,24.41 131.65,24.74
S$234
  Bottom 0: 131.65,24.74 131.44,25.02
S$235
  Bottom 0: 131.44,25.02 131.17,25.25
S$236
  Bottom 0: 131.17,25.25 130.86,25.4
S$237
  Bottom 0: 130.86,25.4 130.51,25.46
S$238
  Bottom 0: 130.51,25.46 130.16,25.44
S$239
  Bottom 0: 130.16,25.44 129.83,25.33
S$240
  Bottom 0: 129.83,25.33 129.54,25.14
S$241
  Bottom 0: 129.54,25.14 129.3,24.89
S$242
  Bottom 0: 129.3,24.89 129.13,24.58
S$243
  Bottom 0: 129.13,24.58 129.04,24.24
S$244
  Bottom 0: 129.04,24.24 129.04,23.89
S$245
  Bottom 0: 129.04,23.89 129.13,23.55
S$246
  Bottom 0: 129.13,23.55 129.18,23.45
S$247
  Bottom 0: 129.18,23.45 126.05,20.32
S$248
  Bottom 0: 126.05,20.32 124.77,20.32
S$249
  Bottom 0: 124.77,20.32 124.82,20.35
S$250
  Bottom 0: 124.82,20.35 125.09,20.57
S$251
  Bottom 0: 125.09,20.57 125.3,20.86
S$252
  Bottom 0: 125.3,20.86 125.42,21.18
S$253
  Bottom 0: 125.42,21.18 125.47,21.53
S$254
  Bottom 0: 125.47,21.53 125.42,21.87
S$255
  Bottom 0: 125.42,21.87 125.3,22.2
S$256
  Bottom 0: 125.3,22.2 125.09,22.48
S$257
  Bottom 0: 125.09,22.48 124.82,22.7
S$258
  Bottom 0: 124.82,22.7 124.51,22.86
S$259
  Bottom 0: 124.51,22.86 124.16,22.92
S$260
  Bottom 0: 124.16,22.92 123.81,22.9
S$261
  Bottom 0: 123.81,22.9 123.48,22.79
S$262
  Bottom 0: 123.48,22.79 123.19,22.6
S$263
  Bottom 0: 123.19,22.6 122.95,22.35
S$264
  Bottom 0: 122.95,22.35 122.78,22.04
S$265
  Bottom 0: 122.78,22.04 122.69,21.7
S$266
  Bottom 0: 122.69,21.7 122.69,21.35
S$267
  Bottom 0: 122.69,21.35 122.78,21.01
S$268
  Bottom 0: 122.78,21.01 122.95,20.7
S$269
  Bottom 0: 122.95,20.7 123.19,20.45
S$270
  Bottom 0: 123.19,20.45 123.39,20.32
S$271
  Bottom 0: 123.39,20.32 122.9,20.32
S$272
  Bottom 0: 122.9,20.32 116.34,26.88
S$273
  Bottom 0: 116.34,26.88 116.34,29.98
S$274
  Bottom 0: 116.34,29.98 116.36,29.96
S$275
  Bottom 0: 116.36,29.96 116.59,29.77
S$276
  Bottom 0: 116.59,29.77 116.87,29.66
S$277
  Bottom 0: 116.87,29.66 117.18,29.64
S$278
  Bottom 0: 117.18,29.64 117.47,29.7
S$279
  Bottom 0: 117.47,29.7 117.68,29.82
S$280
  Bottom 0: 117.68,29.82 135.58,29.82
S$281
  Bottom 0: 135.58,29.82 135.64,29.77
S$282
  Bottom 0: 135.64,29.77 135.92,29.66
S$283
  Bottom 0: 135.92,29.66 136.23,29.64
S$284
  Bottom 0: 136.23,29.64 136.52,29.7
S$285
  Bottom 0: 136.52,29.7 136.79,29.86
S$286
  Bottom 0: 136.79,29.86 136.99,30.08
S$287
  Bottom 0: 136.99,30.08 137.12,30.35
S$288
  Bottom 0: 137.12,30.35 137.17,30.65
S$289
  Bottom 0: 137.17,30.65 137.12,30.95
S$290
  Bottom 0: 137.12,30.95 136.99,31.22
S$291
  Bottom 0: 136.99,31.22 136.85,31.38
S$292
  Bottom 0: 136.85,31.38 137.44,31.38
S$293
  Bottom 0: 137.44,31.38 141.86,26.95
S$294
  Bottom 0: 141.86,26.95 141.86,23.69
S$295
  Bottom 0: 141.86,23.69 134.01,15.84
S$296
  Bottom 0: 134.01,15.84 134.02,15.89
S$297
  Bottom 0: 134.02,15.89 133.97,16.21
S$298
  Bottom 0: 133.97,16.21 133.84,16.51
S$299
  Bottom 0: 133.84,16.51 133.64,16.76
S$300
  Bottom 0: 133.64,16.76 133.37,16.95
S$301
  Bottom 0: 133.37,16.95 133.07,17.06
S$302
  Bottom 0: 133.07,17.06 132.74,17.08
S$303
  Bottom 0: 132.74,17.08 132.42,17.01
S$304
  Bottom 0: 132.42,17.01 132.13,16.86
S$305
  Bottom 0: 132.13,16.86 131.9,16.64
S$306
  Bottom 0: 131.9,16.64 131.73,16.36
S$307
  Bottom 0: 131.73,16.36 131.64,16.05
S$308
  Bottom 0: 131.64,16.05 131.64,15.72
S$309
  Bottom 0: 131.64,15.72 131.73,15.41
S$310
  Bottom 0: 131.73,15.41 131.9,15.14
S$311
  Bottom 0: 131.9,15.14 132.13,14.91
S$312
  Bottom 0: 132.13,14.91 132.42,14.77
S$313
  Bottom 0: 132.42,14.77 132.74,14.7
S$314
  Bottom 0: 132.74,14.7 132.88,14.71
S$315
  Bottom 0: 132.88,14.71 131.38,13.21
S$316
  Bottom 0: 131.38,13.21 131.26,13.21
S$317
  Bottom 0: 131.26,13.21 131.23,13.26
S$318
  Bottom 0: 131.23,13.26 131.02,13.5
S$319
  Bottom 0: 131.02,13.5 130.75,13.68
S$320
  Bottom 0: 130.75,13.68 130.44,13.77
S$321
  Bottom 0: 130.44,13.77 130.11,13.77
S$322
  Bottom 0: 130.11,13.77 129.8,13.68
S$323
  Bottom 0: 129.8,13.68 129.53,13.5
S$324
  Bottom 0: 129.53,13.5 129.31,13.26
S$325
  Bottom 0: 129.31,13.26 129.18,12.96
S$326
  Bottom 0: 129.18,12.96 129.13,12.64
S$327
  Bottom 0: 129.13,12.64 129.18,12.32
S$328
  Bottom 0: 129.18,12.32 129.31,12.02
S$329
  Bottom 0: 129.31,12.02 129.53,11.77
S$330
  Bottom 0: 129.53,11.77 129.8,11.6
S$331
  Bottom 0: 129.8,11.6 130.11,11.5
S$332
  Bottom 0: 130.11,11.5 130.44,11.5
S$333
  Bottom 0: 130.44,11.5 130.75,11.6
S$334
  Bottom 0: 130.75,11.6 131.02,11.77
S$335
  Bottom 0: 131.02,11.77 131.23,12.02
S$336
  Bottom 0: 131.23,12.02 131.26,12.07
S$337
  Bottom 0: 131.26,12.07 131.61,12.07
S$338
  Bottom 0: 131.61,12.07 131.71,12.07
S$339
  Bottom 0: 131.71,12.07 131.79,12.09
S$340
  Bottom 0: 131.79,12.09 131.87,12.13
S$341
  Bottom 0: 131.87,12.13 131.95,12.17
S$342
  Bottom 0: 131.95,12.17 132.02,12.23
S$343
  Bottom 0: 132.02,12.23 141.84,22.05
S$344
  Bottom 0: 141.84,22.05 141.83,22.04
S$345
  Bottom 0: 141.83,22.04 141.74,21.7
S$346
  Bottom 0: 141.74,21.7 141.74,21.35
S$347
  Bottom 0: 141.74,21.35 141.83,21.01
S$348
  Bottom 0: 141.83,21.01 142,20.7
S$349
  Bottom 0: 142,20.7 142.24,20.45
S$350
  Bottom 0: 142.24,20.45 142.53,20.26
S$351
  Bottom 0: 142.53,20.26 142.86,20.16
S$352
  Bottom 0: 142.86,20.16 143.21,20.14
S$353
  Bottom 0: 143.21,20.14 143.56,20.2
S$354
  Bottom 0: 143.56,20.2 143.87,20.35
S$355
  Bottom 0: 143.87,20.35 144.14,20.57
S$356
  Bottom 0: 144.14,20.57 144.35,20.86
S$357
  Bottom 0: 144.35,20.86 144.47,21.18
S$358
  Bottom 0: 144.47,21.18 144.52,21.53
S$359
  Bottom 0: 144.52,21.53 144.47,21.87
S$360
  Bottom 0: 144.47,21.87 144.35,22.2
S$361
  Bottom 0: 144.35,22.2 144.14,22.48
S$362
  Bottom 0: 144.14,22.48 143.87,22.7
S$363
  Bottom 0: 143.87,22.7 143.56,22.86
S$364
  Bottom 0: 143.56,22.86 143.21,22.92
S$365
  Bottom 0: 143.21,22.92 142.86,22.9
S$366
  Bottom 0: 142.86,22.9 142.59,22.81
S$367
  Bottom 0: 142.59,22.81 142.83,23.05
S$368
  Bottom 0: 142.83,23.05 142.89,23.12
S$369
  Bottom 0: 142.89,23.12 142.94,23.19
S$370
  Bottom 0: 142.94,23.19 142.97,23.27
S$371
  Bottom 0: 142.97,23.27 142.99,23.36
S$372
  Bottom 0: 142.99,23.36 143,23.45
S$373
  Bottom 0: 143,23.45 143,26.95
S$374
  Bottom 0: 143,26.95 143.58,27.53
S$375
  Bottom 0: 143.58,27.53 143.55,27.48
S$376
  Bottom 0: 143.55,27.48 143.42,27.05
S$377
  Bottom 0: 143.42,27.05 143.38,26.61
S$378
  Bottom 0: 143.38,26.61 143.42,26.16
S$379
  Bottom 0: 143.42,26.16 143.55,25.73
S$380
  Bottom 0: 143.55,25.73 143.77,25.34
S$381
  Bottom 0: 143.77,25.34 144.05,24.99
S$382
  Bottom 0: 144.05,24.99 144.4,24.71
S$383
  Bottom 0: 144.4,24.71 144.79,24.49
S$384
  Bottom 0: 144.79,24.49 145.22,24.37
S$385
  Bottom 0: 145.22,24.37 145.67,24.32
S$386
  Bottom 0: 145.67,24.32 146.11,24.37
S$387
  Bottom 0: 146.11,24.37 146.54,24.49
S$388
  Bottom 0: 146.54,24.49 146.94,24.71
S$389
  Bottom 0: 146.94,24.71 147.28,24.99
S$390
  Bottom 0: 147.28,24.99 147.41,25.14
S$391
  Bottom 0: 147.41,25.14 147.41,20.24
S$392
  Bottom 0: 147.41,20.24 147.38,20.22
S$393
  Bottom 0: 147.38,20.22 133.43,6.26
S$394
  Bottom 0: 133.43,6.26 133.25,6.35
S$395
  Bottom 0: 133.25,6.35 132.9,6.41
S$396
  Bottom 0: 132.9,6.41 132.55,6.39
S$397
  Bottom 0: 132.55,6.39 132.22,6.28
S$398
  Bottom 0: 132.22,6.28 131.93,6.09
S$399
  Bottom 0: 131.93,6.09 131.69,5.84
S$400
  Bottom 0: 131.69,5.84 131.51,5.53
S$401
  Bottom 0: 131.51,5.53 131.43,5.19
S$402
  Bottom 0: 131.43,5.19 131.43,4.84
S$403
  Bottom 0: 131.43,4.84 131.51,4.5
S$404
  Bottom 0: 131.51,4.5 131.69,4.19
S$405
  Bottom 0: 131.69,4.19 131.93,3.94
S$406
  Bottom 0: 131.93,3.94 132.22,3.75
S$407
  Bottom 0: 132.22,3.75 132.55,3.65
S$408
  Bottom 0: 132.55,3.65 132.9,3.62
S$409
  Bottom 0: 132.9,3.62 133.25,3.69
S$410
  Bottom 0: 133.25,3.69 133.56,3.84
S$411
  Bottom 0: 133.56,3.84 133.83,4.06
S$412
  Bottom 0: 133.83,4.06 134.04,4.35
S$413
  Bottom 0: 134.04,4.35 134.16,4.67
S$414
  Bottom 0: 134.16,4.67 134.21,5.02
S$415
  Bottom 0: 134.21,5.02 134.16,5.36
S$416
  Bottom 0: 134.16,5.36 134.06,5.63
S$417
  Bottom 0: 134.06,5.63 147.88,19.46
S$418
  Bottom 0: 147.88,19.46 164.36,19.46
S$419
  Bottom 0: 164.36,19.46 164.43,19.46
S$420
  Bottom 0: 164.43,19.46 164.5,19.48
S$421
  Bottom 0: 164.5,19.48 164.56,19.5
S$422
  Bottom 0: 164.56,19.5 164.62,19.55
S$423
  Bottom 0: 164.62,19.55 164.68,19.59
S$424
  Bottom 0: 164.68,19.59 167.91,22.82
S$425
  Bottom 0: 167.91,22.82 167.93,22.8
S$426
  Bottom 0: 167.93,22.8 168.26,22.7
S$427
  Bottom 0: 168.26,22.7 168.61,22.68
S$428
  Bottom 0: 168.61,22.68 168.96,22.74
S$429
  Bottom 0: 168.96,22.74 169.27,22.89
S$430
  Bottom 0: 169.27,22.89 169.54,23.11
S$431
  Bottom 0: 169.54,23.11 169.72,23.36
S$432
  Bottom 0: 169.72,23.36 169.72,14.76
S$433
  Bottom 0: 169.72,14.76 167.57,12.6
S$434
  Bottom 0: 167.57,12.6 167.7,12.91
S$435
  Bottom 0: 167.7,12.91 167.83,13.4
S$436
  Bottom 0: 167.83,13.4 167.87,13.92
S$437
  Bottom 0: 167.87,13.92 167.83,14.44
S$438
  Bottom 0: 167.83,14.44 167.7,14.94
S$439
  Bottom 0: 167.7,14.94 167.5,15.41
S$440
  Bottom 0: 167.5,15.41 167.21,15.85
S$441
  Bottom 0: 167.21,15.85 166.86,16.23
S$442
  Bottom 0: 166.86,16.23 166.45,16.55
S$443
  Bottom 0: 166.45,16.55 166,16.79
S$444
  Bottom 0: 166,16.79 165.5,16.96
S$445
  Bottom 0: 165.5,16.96 165,17.05
S$446
  Bottom 0: 165,17.05 164.47,17.05
S$447
  Bottom 0: 164.47,17.05 163.97,16.96
S$448
  Bottom 0: 163.97,16.96 163.48,16.79
S$449
  Bottom 0: 163.48,16.79 163.03,16.55
S$450
  Bottom 0: 163.03,16.55 162.61,16.23
S$451
  Bottom 0: 162.61,16.23 162.26,15.85
S$452
  Bottom 0: 162.26,15.85 161.98,15.41
S$453
  Bottom 0: 161.98,15.41 161.77,14.94
S$454
  Bottom 0: 161.77,14.94 161.64,14.44
S$455
  Bottom 0: 161.64,14.44 161.6,13.92
S$456
  Bottom 0: 161.6,13.92 161.64,13.4
S$457
  Bottom 0: 161.64,13.4 161.77,12.91
S$458
  Bottom 0: 161.77,12.91 161.98,12.43
S$459
  Bottom 0: 161.98,12.43 162.26,12
S$460
  Bottom 0: 162.26,12 162.61,11.62
S$461
  Bottom 0: 162.61,11.62 163.03,11.29
S$462
  Bottom 0: 163.03,11.29 163.48,11.05
S$463
  Bottom 0: 163.48,11.05 163.97,10.88
S$464
  Bottom 0: 163.97,10.88 164.47,10.8
S$465
  Bottom 0: 164.47,10.8 165,10.8
S$466
  Bottom 0: 165,10.8 165.5,10.88
S$467
  Bottom 0: 165.5,10.88 166,11.05
S$468
  Bottom 0: 166,11.05 166.05,11.08
S$469
  Bottom 0: 166.05,11.08 163.65,8.68
S$470
  Bottom 0: 163.65,8.68 163.39,8.7
S$471
  Bottom 0: 163.39,8.7 163.06,8.63
S$472
  Bottom 0: 163.06,8.63 162.78,8.49
S$473
  Bottom 0: 162.78,8.49 162.54,8.26
S$474
  Bottom 0: 162.54,8.26 162.37,7.99
S$475
  Bottom 0: 162.37,7.99 162.28,7.67
S$476
  Bottom 0: 162.28,7.67 162.28,7.35
S$477
  Bottom 0: 162.28,7.35 162.37,7.03
S$478
  Bottom 0: 162.37,7.03 162.54,6.76
S$479
  Bottom 0: 162.54,6.76 162.78,6.54
S$480
  Bottom 0: 162.78,6.54 163.06,6.39
S$481
  Bottom 0: 163.06,6.39 163.39,6.32
S$482
  Bottom 0: 163.39,6.32 163.71,6.34
S$483
  Bottom 0: 163.71,6.34 164.01,6.45
S$484
  Bottom 0: 164.01,6.45 164.28,6.64
S$485
  Bottom 0: 164.28,6.64 164.49,6.89
S$486
  Bottom 0: 164.49,6.89 164.62,7.19
S$487
  Bottom 0: 164.62,7.19 164.66,7.51
S$488
  Bottom 0: 164.66,7.51 164.62,7.83
S$489
  Bottom 0: 164.62,7.83 164.55,7.98
S$490
  Bottom 0: 164.55,7.98 164.81,8.23
S$491
  Bottom 0: 164.81,8.23 164.81,6.57
S$492
  Bottom 0: 164.81,6.57 164.82,6.5
S$493
  Bottom 0: 164.82,6.5 164.86,6.42
S$494
  Bottom 0: 164.86,6.42 164.91,6.37
S$495
  Bottom 0: 164.91,6.37 164.98,6.33
S$496
  Bottom 0: 164.98,6.33 165.06,6.32
S$497
  Bottom 0: 165.06,6.32 166.94,6.32
S$498
  Bottom 0: 166.94,6.32 167.02,6.33
S$499
  Bottom 0: 167.02,6.33 167.09,6.37
S$500
  Bottom 0: 167.09,6.37 167.15,6.42
S$501
  Bottom 0: 167.15,6.42 167.19,6.5
S$502
  Bottom 0: 167.19,6.5 167.2,6.57
S$503
  Bottom 0: 167.2,6.57 167.2,8.45
S$504
  Bottom 0: 167.2,8.45 167.19,8.53
S$505
  Bottom 0: 167.19,8.53 167.15,8.6
S$506
  Bottom 0: 167.15,8.6 167.09,8.65
S$507
  Bottom 0: 167.09,8.65 167.02,8.69
S$508
  Bottom 0: 167.02,8.69 166.94,8.71
S$509
  Bottom 0: 166.94,8.71 165.28,8.71
S$510
  Bottom 0: 165.28,8.71 170.7,14.12
S$511
  Bottom 0: 170.7,14.12 170.76,14.19
S$512
  Bottom 0: 170.76,14.19 170.8,14.26
S$513
  Bottom 0: 170.8,14.26 170.84,14.34
S$514
  Bottom 0: 170.84,14.34 170.86,14.43
S$515
  Bottom 0: 170.86,14.43 170.86,14.52
S$516
  Bottom 0: 170.86,14.52 170.86,26.81
S$517
  Bottom 0: 170.86,26.81 173.5,26.81
S$518
  Bottom 0: 173.5,26.81 173.59,26.82
S$519
  Bottom 0: 173.59,26.82 173.68,26.84
S$520
  Bottom 0: 173.68,26.84 173.76,26.87
S$521
  Bottom 0: 173.76,26.87 173.84,26.92
S$522
  Bottom 0: 173.84,26.92 173.9,26.98
S$523
  Bottom 0: 173.9,26.98 177.1,30.18
S$524
  Bottom 0: 177.1,30.18 177.26,30.22
S$525
  Bottom 0: 177.26,30.22 177.41,30.33
S$526
  Bottom 0: 177.41,30.33 177.41,8.55
S$527
  Bottom 0: 177.41,8.55 177.28,8.49
S$528
  Bottom 0: 177.28,8.49 177.05,8.26
S$529
  Bottom 0: 177.05,8.26 176.88,7.99
S$530
  Bottom 0: 176.88,7.99 176.79,7.67
S$531
  Bottom 0: 176.79,7.67 176.79,7.35
S$532
  Bottom 0: 176.79,7.35 176.88,7.03
S$533
  Bottom 0: 176.88,7.03 177.05,6.76
S$534
  Bottom 0: 177.05,6.76 177.28,6.54
S$535
  Bottom 0: 177.28,6.54 177.57,6.39
S$536
  Bottom 0: 177.57,6.39 177.89,6.32
S$537
  Bottom 0: 177.89,6.32 178.22,6.34
S$538
  Bottom 0: 178.22,6.34 178.52,6.45
S$539
  Bottom 0: 178.52,6.45 178.79,6.64
S$540
  Bottom 0: 178.79,6.64 179,6.89
S$541
  Bottom 0: 179,6.89 179.12,7.19
S$542
  Bottom 0: 179.12,7.19 179.17,7.51
S$543
  Bottom 0: 179.17,7.51 179.12,7.83
S$544
  Bottom 0: 179.12,7.83 179,8.13
S$545
  Bottom 0: 179,8.13 178.79,8.38
S$546
  Bottom 0: 178.79,8.38 178.54,8.56
S$547
  Bottom 0: 178.54,8.56 178.54,32.64
S$548
  Bottom 0: 178.54,32.64 178.64,32.74
S$549
  Bottom 0: 178.64,32.74 181.42,32.74
S$550
  Bottom 0: 181.42,32.74 181.4,32.72
S$551
  Bottom 0: 181.4,32.72 181.36,32.65
S$552
  Bottom 0: 181.36,32.65 181.35,32.58
S$553
  Bottom 0: 181.35,32.58 181.35,30.8
S$554
  Bottom 0: 181.35,30.8 181.36,30.72
S$555
  Bottom 0: 181.36,30.72 181.4,30.65
S$556
  Bottom 0: 181.4,30.65 181.46,30.59
S$557
  Bottom 0: 181.46,30.59 181.53,30.55
S$558
  Bottom 0: 181.53,30.55 181.61,30.54
S$559
  Bottom 0: 181.61,30.54 183.38,30.54
S$560
  Bottom 0: 183.38,30.54 183.46,30.55
S$561
  Bottom 0: 183.46,30.55 183.53,30.59
S$562
  Bottom 0: 183.53,30.59 183.59,30.65
S$563
  Bottom 0: 183.59,30.65 183.63,30.72
S$564
  Bottom 0: 183.63,30.72 183.64,30.8
S$565
  Bottom 0: 183.64,30.8 183.64,32.58
S$566
  Bottom 0: 183.64,32.58 183.63,32.65
S$567
  Bottom 0: 183.63,32.65 183.59,32.72
S$568
  Bottom 0: 183.59,32.72 183.57,32.74
S$569
  Bottom 0: 183.57,32.74 184.6,32.74
S$570
  Bottom 0: 184.6,32.74 184.56,32.73
S$571
  Bottom 0: 184.56,32.73 184.29,32.55
S$572
  Bottom 0: 184.29,32.55 184.08,32.31
S$573
  Bottom 0: 184.08,32.31 183.94,32.01
S$574
  Bottom 0: 183.94,32.01 183.89,31.69
S$575
  Bottom 0: 183.89,31.69 183.94,31.37
S$576
  Bottom 0: 183.94,31.37 184.08,31.07
S$577
  Bottom 0: 184.08,31.07 184.29,30.82
S$578
  Bottom 0: 184.29,30.82 184.56,30.64
S$579
  Bottom 0: 184.56,30.64 184.87,30.55
S$580
  Bottom 0: 184.87,30.55 185.2,30.55
S$581
  Bottom 0: 185.2,30.55 185.51,30.64
S$582
  Bottom 0: 185.51,30.64 185.78,30.82
S$583
  Bottom 0: 185.78,30.82 186,31.07
S$584
  Bottom 0: 186,31.07 186.02,31.12
S$585
  Bottom 0: 186.02,31.12 192.41,31.12
S$586
  Bottom 0: 192.41,31.12 192.39,31.09
S$587
  Bottom 0: 192.39,31.09 191.89,31.09
S$588
  Bottom 0: 191.89,31.09 191.82,31.09
S$589
  Bottom 0: 191.82,31.09 191.75,31.07
S$590
  Bottom 0: 191.75,31.07 191.69,31.05
S$591
  Bottom 0: 191.69,31.05 191.63,31.01
S$592
  Bottom 0: 191.63,31.01 191.57,30.96
S$593
  Bottom 0: 191.57,30.96 185.38,24.77
S$594
  Bottom 0: 185.38,24.77 185.34,24.71
S$595
  Bottom 0: 185.34,24.71 185.3,24.65
S$596
  Bottom 0: 185.3,24.65 185.27,24.59
S$597
  Bottom 0: 185.27,24.59 185.25,24.52
S$598
  Bottom 0: 185.25,24.52 185.25,24.45
S$599
  Bottom 0: 185.25,24.45 185.25,16.78
S$600
  Bottom 0: 185.25,16.78 185.18,16.76
S$601
  Bottom 0: 185.18,16.76 184.94,16.57
S$602
  Bottom 0: 184.94,16.57 184.78,16.32
S$603
  Bottom 0: 184.78,16.32 184.68,16.03
S$604
  Bottom 0: 184.68,16.03 184.68,15.72
S$605
  Bottom 0: 184.68,15.72 184.78,15.44
S$606
  Bottom 0: 184.78,15.44 184.94,15.19
S$607
  Bottom 0: 184.94,15.19 185.18,15
S$608
  Bottom 0: 185.18,15 185.46,14.89
S$609
  Bottom 0: 185.46,14.89 185.76,14.87
S$610
  Bottom 0: 185.76,14.87 186.06,14.93
S$611
  Bottom 0: 186.06,14.93 186.33,15.09
S$612
  Bottom 0: 186.33,15.09 186.53,15.3
S$613
  Bottom 0: 186.53,15.3 186.66,15.58
S$614
  Bottom 0: 186.66,15.58 186.71,15.88
S$615
  Bottom 0: 186.71,15.88 186.66,16.18
S$616
  Bottom 0: 186.66,16.18 186.53,16.45
S$617
  Bottom 0: 186.53,16.45 186.33,16.67
S$618
  Bottom 0: 186.33,16.67 186.13,16.78
S$619
  Bottom 0: 186.13,16.78 186.13,24.27
S$620
  Bottom 0: 186.13,24.27 186.22,24.35
S$621
  Bottom 0: 186.22,24.35 186.19,24.24
S$622
  Bottom 0: 186.19,24.24 186.19,23.89
S$623
  Bottom 0: 186.19,23.89 186.27,23.55
S$624
  Bottom 0: 186.27,23.55 186.45,23.24
S$625
  Bottom 0: 186.45,23.24 186.69,22.99
S$626
  Bottom 0: 186.69,22.99 186.98,22.8
S$627
  Bottom 0: 186.98,22.8 187.31,22.7
S$628
  Bottom 0: 187.31,22.7 187.66,22.68
S$629
  Bottom 0: 187.66,22.68 188.01,22.74
S$630
  Bottom 0: 188.01,22.74 188.2,22.83
S$631
  Bottom 0: 188.2,22.83 191.88,19.14
S$632
  Bottom 0: 191.88,19.14 191.94,19.1
S$633
  Bottom 0: 191.94,19.1 192,19.06
S$634
  Bottom 0: 192,19.06 192.06,19.03
S$635
  Bottom 0: 192.06,19.03 192.12,19.02
S$636
  Bottom 0: 192.12,19.02 192.19,19.01
S$637
  Bottom 0: 192.19,19.01 196.56,19.01
S$638
  Bottom 0: 196.56,19.01 201.81,13.77
S$639
  Bottom 0: 201.81,13.77 201.55,13.77
S$640
  Bottom 0: 201.55,13.77 201.24,13.68
S$641
  Bottom 0: 201.24,13.68 200.96,13.5
S$642
  Bottom 0: 200.96,13.5 200.75,13.26
S$643
  Bottom 0: 200.75,13.26 200.61,12.96
S$644
  Bottom 0: 200.61,12.96 200.57,12.64
S$645
  Bottom 0: 200.57,12.64 200.61,12.32
S$646
  Bottom 0: 200.61,12.32 200.75,12.02
S$647
  Bottom 0: 200.75,12.02 200.96,11.77
S$648
  Bottom 0: 200.96,11.77 201.24,11.6
S$649
  Bottom 0: 201.24,11.6 201.55,11.5
S$650
  Bottom 0: 201.55,11.5 201.87,11.5
S$651
  Bottom 0: 201.87,11.5 202.18,11.6
S$652
  Bottom 0: 202.18,11.6 202.46,11.77
S$653
  Bottom 0: 202.46,11.77 202.67,12.02
S$654
  Bottom 0: 202.67,12.02 202.81,12.32
S$655
  Bottom 0: 202.81,12.32 202.85,12.64
S$656
  Bottom 0: 202.85,12.64 202.84,12.74
S$657
  Bottom 0: 202.84,12.74 203.81,11.77
S$658
  Bottom 0: 203.81,11.77 203.81,6.33
S$659
  Bottom 0: 203.81,6.33 203.66,6.28
S$660
  Bottom 0: 203.66,6.28 203.36,6.09
S$661
  Bottom 0: 203.36,6.09 203.12,5.84
S$662
  Bottom 0: 203.12,5.84 202.95,5.53
S$663
  Bottom 0: 202.95,5.53 202.86,5.19
S$664
  Bottom 0: 202.86,5.19 202.86,4.84
S$665
  Bottom 0: 202.86,4.84 202.95,4.5
S$666
  Bottom 0: 202.95,4.5 203.12,4.19
S$667
  Bottom 0: 203.12,4.19 203.36,3.94
S$668
  Bottom 0: 203.36,3.94 203.66,3.75
S$669
  Bottom 0: 203.66,3.75 203.98,3.65
S$670
  Bottom 0: 203.98,3.65 204.34,3.62
S$671
  Bottom 0: 204.34,3.62 204.68,3.69
S$672
  Bottom 0: 204.68,3.69 204.86,3.77
S$673
  Bottom 0: 204.86,3.77 206.13,2.51
S$674
  Bottom 0: 206.13,2.51 206.19,2.47
S$675
  Bottom 0: 206.19,2.47 206.25,2.43
S$676
  Bottom 0: 206.25,2.43 206.31,2.4
S$677
  Bottom 0: 206.31,2.4 206.37,2.38
S$678
  Bottom 0: 206.37,2.38 206.44,2.38
S$679
  Bottom 0: 206.44,2.38 215.8,2.38
S$680
  Bottom 0: 215.8,2.38 215.87,2.38
S$681
  Bottom 0: 215.87,2.38 215.94,2.4
S$682
  Bottom 0: 215.94,2.4 216,2.43
S$683
  Bottom 0: 216,2.43 216.06,2.47
S$684
  Bottom 0: 216.06,2.47 216.11,2.51
S$685
  Bottom 0: 216.11,2.51 217.23,3.63
S$686
  Bottom 0: 217.23,3.63 220.94,3.63
S$687
  Bottom 0: 220.94,3.63 220.82,3.55
S$688
  Bottom 0: 220.82,3.55 220.58,3.3
S$689
  Bottom 0: 220.58,3.3 220.41,2.99
S$690
  Bottom 0: 220.41,2.99 220.32,2.65
S$691
  Bottom 0: 220.32,2.65 220.32,2.3
S$692
  Bottom 0: 220.32,2.3 220.41,1.96
S$693
  Bottom 0: 220.41,1.96 220.58,1.65
S$694
  Bottom 0: 220.58,1.65 220.82,1.4
S$695
  Bottom 0: 220.82,1.4 221.12,1.21
S$696
  Bottom 0: 221.12,1.21 221.44,1.1
S$697
  Bottom 0: 221.44,1.1 221.79,1.08
S$698
  Bottom 0: 221.79,1.08 222.14,1.15
S$699
  Bottom 0: 222.14,1.15 222.46,1.3
S$700
  Bottom 0: 222.46,1.3 222.72,1.52
S$701
  Bottom 0: 222.72,1.52 222.93,1.81
S$702
  Bottom 0: 222.93,1.81 223.06,2.13
S$703
  Bottom 0: 223.06,2.13 223.1,2.48
S$704
  Bottom 0: 223.1,2.48 223.06,2.82
S$705
  Bottom 0: 223.06,2.82 222.93,3.15
S$706
  Bottom 0: 222.93,3.15 222.72,3.43
S$707
  Bottom 0: 222.72,3.43 222.49,3.63
S$708
  Bottom 0: 222.49,3.63 224.15,3.63
S$709
  Bottom 0: 224.15,3.63 224.66,3.12
S$710
  Bottom 0: 224.66,3.12 224.72,3.08
S$711
  Bottom 0: 224.72,3.08 224.78,3.04
S$712
  Bottom 0: 224.78,3.04 224.84,3.02
S$713
  Bottom 0: 224.84,3.02 224.9,3
S$714
  Bottom 0: 224.9,3 224.97,3
S$715
  Bottom 0: 224.97,3 228.62,3
S$716
  Bottom 0: 228.62,3 228.69,3
S$717
  Bottom 0: 228.69,3 228.75,3.02
S$718
  Bottom 0: 228.75,3.02 228.81,3.04
S$719
  Bottom 0: 228.81,3.04 228.87,3.08
S$720
  Bottom 0: 228.87,3.08 228.93,3.12
S$721
  Bottom 0: 228.93,3.12 237.55,11.74
S$722
  Bottom 0: 237.55,11.74 237.55,11.44
S$723
  Bottom 0: 237.55,11.44 237.64,11.15
S$724
  Bottom 0: 237.64,11.15 237.81,10.9
S$725
  Bottom 0: 237.81,10.9 238.05,10.72
S$726
  Bottom 0: 238.05,10.72 238.33,10.6
S$727
  Bottom 0: 238.33,10.6 238.64,10.58
S$728
  Bottom 0: 238.64,10.58 238.88,10.64
S$729
  Bottom 0: 238.88,10.64 245.67,3.86
S$730
  Bottom 0: 245.67,3.86 245.61,3.87
S$731
  Bottom 0: 245.61,3.87 245.26,3.85
S$732
  Bottom 0: 245.26,3.85 244.93,3.74
S$733
  Bottom 0: 244.93,3.74 244.9,3.73
S$734
  Bottom 0: 244.9,3.73 244.34,4.29
S$735
  Bottom 0: 244.34,4.29 244.28,4.33
S$736
  Bottom 0: 244.28,4.33 244.22,4.37
S$737
  Bottom 0: 244.22,4.37 244.16,4.4
S$738
  Bottom 0: 244.16,4.4 244.1,4.41
S$739
  Bottom 0: 244.1,4.41 244.03,4.42
S$740
  Bottom 0: 244.03,4.42 239.46,4.42
S$741
  Bottom 0: 239.46,4.42 239.4,4.55
S$742
  Bottom 0: 239.4,4.55 239.19,4.77
S$743
  Bottom 0: 239.19,4.77 238.93,4.92
S$744
  Bottom 0: 238.93,4.92 238.64,4.99
S$745
  Bottom 0: 238.64,4.99 238.33,4.97
S$746
  Bottom 0: 238.33,4.97 238.05,4.85
S$747
  Bottom 0: 238.05,4.85 237.81,4.67
S$748
  Bottom 0: 237.81,4.67 237.64,4.42
S$749
  Bottom 0: 237.64,4.42 237.55,4.13
S$750
  Bottom 0: 237.55,4.13 237.55,3.82
S$751
  Bottom 0: 237.55,3.82 237.64,3.53
S$752
  Bottom 0: 237.64,3.53 237.81,3.28
S$753
  Bottom 0: 237.81,3.28 238.05,3.1
S$754
  Bottom 0: 238.05,3.1 238.33,2.98
S$755
  Bottom 0: 238.33,2.98 238.64,2.96
S$756
  Bottom 0: 238.64,2.96 238.93,3.03
S$757
  Bottom 0: 238.93,3.03 239.19,3.18
S$758
  Bottom 0: 239.19,3.18 239.4,3.4
S$759
  Bottom 0: 239.4,3.4 239.46,3.53
S$760
  Bottom 0: 239.46,3.53 243.84,3.53
S$761
  Bottom 0: 243.84,3.53 244.28,3.09
S$762
  Bottom 0: 244.28,3.09 244.22,2.99
S$763
  Bottom 0: 244.22,2.99 244.14,2.65
S$764
  Bottom 0: 244.14,2.65 244.14,2.3
S$765
  Bottom 0: 244.14,2.3 244.22,1.96
S$766
  Bottom 0: 244.22,1.96 244.4,1.65
S$767
  Bottom 0: 244.4,1.65 244.63,1.4
S$768
  Bottom 0: 244.63,1.4 244.93,1.21
S$769
  Bottom 0: 244.93,1.21 245.26,1.1
S$770
  Bottom 0: 245.26,1.1 245.61,1.08
S$771
  Bottom 0: 245.61,1.08 245.96,1.15
S$772
  Bottom 0: 245.96,1.15 246.27,1.3
S$773
  Bottom 0: 246.27,1.3 246.54,1.52
S$774
  Bottom 0: 246.54,1.52 246.75,1.81
S$775
  Bottom 0: 246.75,1.81 246.88,2.13
S$776
  Bottom 0: 246.88,2.13 246.92,2.48
S$777
  Bottom 0: 246.92,2.48 246.88,2.82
